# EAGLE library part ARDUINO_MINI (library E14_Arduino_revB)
Device for representing an Arduino Mini board with a footprint in an EAGLE design. Created by Dave Young for Element14. More EAGLE documentation at: http://www.element14.com/community/community/knode/cadsoft_eagle
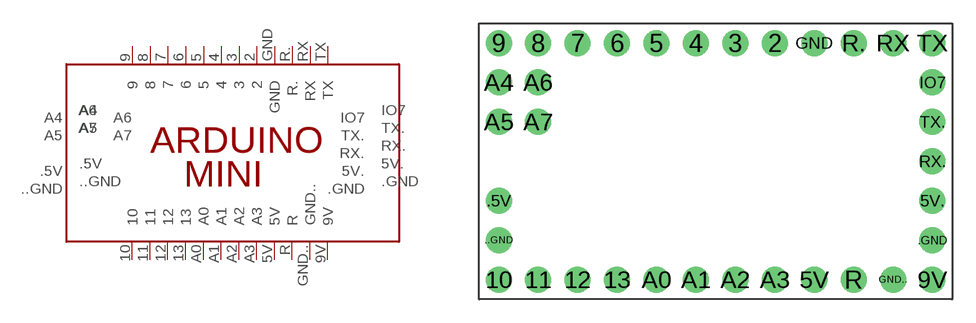
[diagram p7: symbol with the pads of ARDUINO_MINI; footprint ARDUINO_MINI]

Designator prefix PCB

## ARDUINO_MINI  [ARDUINO_MINI]
2  2
3  3
4  4
5  5
5V  5V
5V.  5V.
6  6
7  7
8  8
9  9
9V  9V
10  10
11  11
12  12
13  13
.5V  .5V
..GND  ..GND
.GND  .GND
A0  A0
A1  A1
A2  A2
A3  A3
A4  A4
A5  A5
A6  A6
A7  A7
GND  GND
GND..  GND..
IO7  IO7
R  R
R.  R.
RX  RX
RX.  RX.
TX  TX
TX.  TX.

## Footprint ARDUINO_MINI (pad centres in mm)
Footprint for representing an Arduino Mini board in an EAGLE schematic. Created by Dave Young for Element14. More EAGLE documentation at: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
drill 1.016 pad 1.676: 2 19.05,16.51; 3 16.51,16.51; 4 13.97,16.51; 5 11.43,16.51; 5V 21.59,1.27; 5V. 29.21,6.35; 6 8.89,16.51; 7 6.35,16.51; 8 3.81,16.51; 9 1.27,16.51; 9V 29.21,1.27; 10 1.27,1.27; 11 3.81,1.27; 12 6.35,1.27; 13 8.89,1.27; .5V 1.27,6.35; ..GND 1.27,3.81; .GND 29.21,3.81; A0 11.43,1.27; A1 13.97,1.27; A2 16.51,1.27; A3 19.05,1.27; A4 1.27,13.97; A5 1.27,11.43; A6 3.81,13.97; A7 3.81,11.43; GND 21.59,16.51; GND.. 26.67,1.27; IO7 29.21,13.97; R 24.13,1.27; R. 24.13,16.51; RX 26.67,16.51; RX. 29.21,8.89; TX 29.21,16.51; TX. 29.21,11.43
